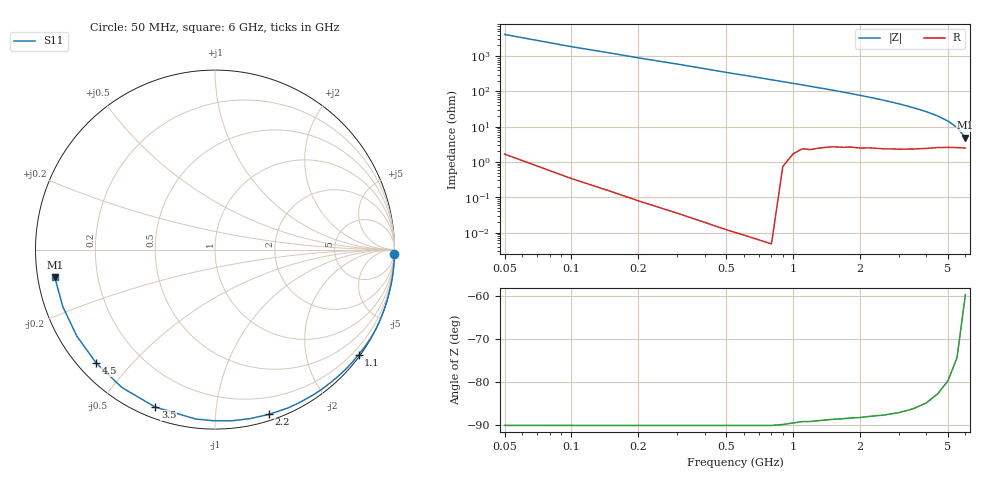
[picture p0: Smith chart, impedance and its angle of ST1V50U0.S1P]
! SIEMENS Discrete & RF Semiconductors
! BA892
! Si PIN Diode in SCD-80
! VR = 1.5 V
! S-Parameters:  September  1997
# GHz  S  MA  R  50
!  f  S11
! GHz  MAG  ANG
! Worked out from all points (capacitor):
!   34 points, 50 MHz to 6 GHz, reference 50 ohm
!   read as one part to ground: C = 861 fF near 50 MHz
!   lowest |Z| = 4.9 ohm at 6 GHz (marker M1)
!   S11 on the Smith chart (normalised r, x): 50 MHz: 0, -82; 1.1 GHz: 0.05, -3.06; 2.2 GHz: 0.05, -1.38; 3.5 GHz: 0.05, -0.69; 4.5 GHz: 0.05, -0.40; 6 GHz: 0.05, -0.08
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0.05  1 -1.4
0.15  1 -4.7
0.25  1 -8.0
0.4  1 -13.0
0.5  1 -16.5
0.6  1 -19.7
0.7  1 -23.0
0.8  1 -26.4
0.9  0.9981 -29.6
1.1  0.9909 -36.2
1.2  0.9897 -39.5
1.3  0.987 -42.8
1.5  0.9815 -49.2
1.6  0.9794 -52.5
1.7  0.9775 -55.8
1.9  0.9729 -62.2
2  0.9713 -65.4
2.2  0.9659 -71.8
2.4  0.962 -78.2
2.6  0.9584 -84.4
2.8  0.9534 -90.6
3  0.95 -96.5
3.5  0.9383 -110.8
4  0.927 -124.0
4.5  0.9151 -136.4
5  0.9083 -148.0
5.5  0.9056 -159.3
6  0.9062 -170.3
